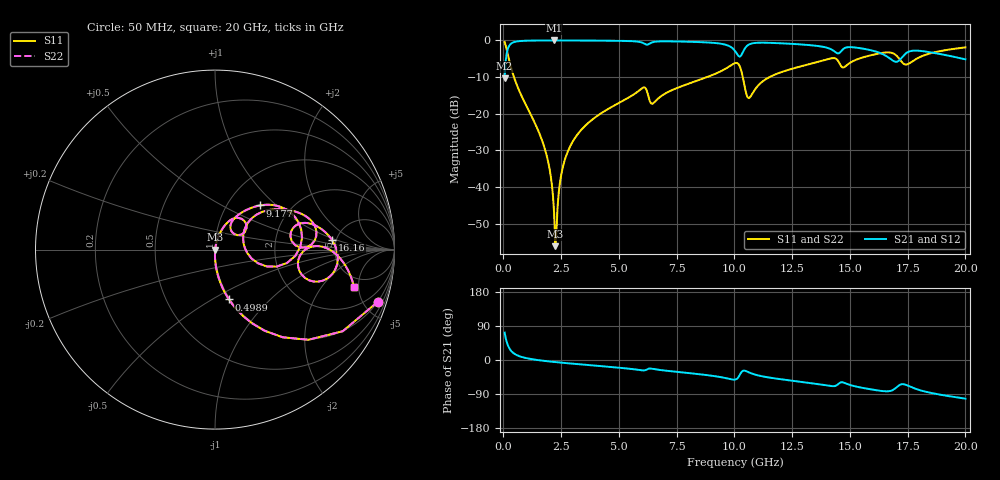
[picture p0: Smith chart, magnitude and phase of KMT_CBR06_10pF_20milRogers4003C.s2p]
! Data measured by Modelithics Inc. support@modelithics.com 813-866-6335
! KEMET CBR0603 10pF, Pad Width= 0.851mm, Pad Length= 0.64mm, Pad Gap= 0.62mm, 20mil Rogers 4003C substrate Data, January 2022
# hz S ma R 50
! 2 Port Network Data from SP1.SP block
! freq  magS11  angS11  magS21  angS21  magS12  angS12  magS22  angS22
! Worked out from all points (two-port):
!   401 points, 50 MHz to 20 GHz, reference 50 ohm
!   highest |S21| = -0.01 dB at 2.195 GHz (marker M1); lowest = -10.4 dB at 50 MHz (marker M2)
!   |S21| within 3 dB of the highest: 159.3 MHz to 10.04 GHz (9.879 GHz wide, 194 % of centre); 10.38 GHz to 14.34 GHz (3.955 GHz wide, 32 % of centre)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
!   lowest |S11| = -56.2 dB at 2.244 GHz (marker M3), VSWR 1.00, Z = 50.1 - j0.108 ohm
!   |S11| at or under -10 dB: 454.6 MHz to 8.822 GHz (8.368 GHz wide, 180 % of centre); 10.36 GHz to 11.52 GHz (1.161 GHz wide, 10.6 % of centre)
!   |S22| runs from -56.2 to -0.4 dB; largest |S21 - S12| = 0
!   S11 on the Smith chart (normalised r, x): 50 MHz: 0.99, -6.27; 498.9 MHz: 0.99, -0.60; 9.177 GHz: 1.41, +0.79; 16.16 GHz: 4.59, +0.88; 20 GHz: 3.73, -4.44
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5e7  0.9532 -17.7  0.3021 72.3  0.3021 72.3  0.9532 -17.7
2.99375e8  0.4599 -63.3  0.8874 26.6  0.8874 26.6  0.4599 -63.3
4.98875e8  0.2883 -74.3  0.9568 15.5  0.9568 15.5  0.2883 -74.3
1.795625e9  0.0328 -90.6  0.9983 -2.5  0.9983 -2.5  0.0328 -90.6
2.045e9  0.01425 -89.5  0.9987 -4.2  0.9987 -4.2  0.01425 -89.5
2.194625e9  0.004332 -79.0  0.9987 -5.2  0.9987 -5.2  0.004332 -79.0
2.2445e9  0.001553 -43.7  0.9987 -5.5  0.9987 -5.5  0.001553 -43.7
2.6435e9  0.02268 78.9  0.9983 -7.8  0.9983 -7.8  0.02268 78.9
3.391625e9  0.0612 76.7  0.9965 -11.8  0.9965 -11.8  0.0612 76.7
6.035e9  0.226 49.6  0.9248 -27.5  0.9248 -27.5  0.226 49.6
6.434e9  0.1361 44.3  0.9394 -23.0  0.9394 -23.0  0.1361 44.3
6.73325e9  0.1646 57.9  0.9684 -25.9  0.9684 -25.9  0.1646 57.9
9.177125e9  0.3506 44.5  0.9207 -42.9  0.9207 -42.9  0.3506 44.5
1.0025e10  0.4898 17.8  0.7172 -51.8  0.7172 -51.8  0.4898 17.8
1.032425e10  0.3571 -15.3  0.6506 -30.6  0.6506 -30.6  0.3571 -15.3
1.06235e10  0.163 12.3  0.8774 -32.5  0.8774 -32.5  0.163 12.3
1.336662e10  0.4857 26.3  0.856 -61.6  0.856 -61.6  0.4857 26.3
1.615962e10  0.6534 4.8  0.6986 -79.9  0.6986 -79.9  0.6534 4.8
1.670825e10  0.685 -6.9  0.5733 -82.1  0.5733 -82.1  0.685 -6.9
1.74065e10  0.4682 -9.2  0.6589 -65.2  0.6589 -65.2  0.4682 -9.2
1.810475e10  0.6067 1.3  0.7167 -81.0  0.7167 -81.0  0.6067 1.3
2e10  0.8032 -15.2  0.5511 -102.0  0.5511 -102.0  0.8032 -15.2
